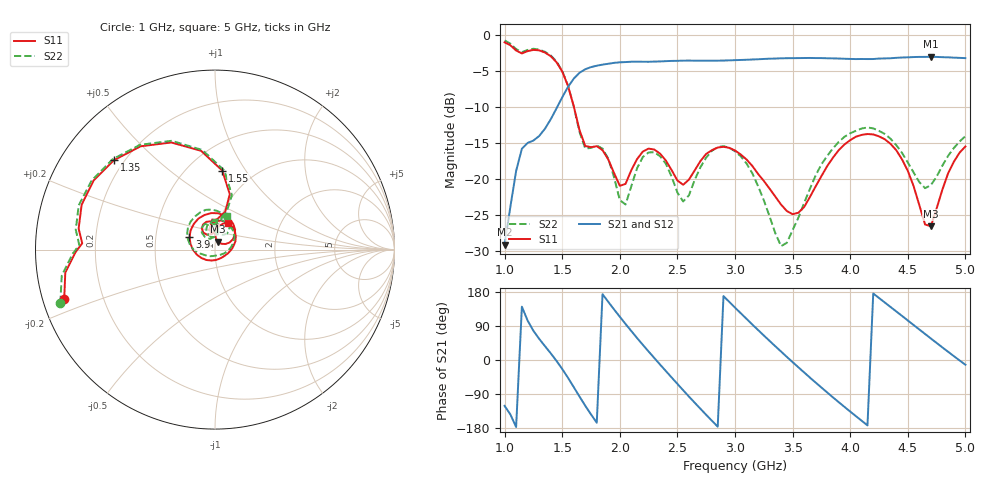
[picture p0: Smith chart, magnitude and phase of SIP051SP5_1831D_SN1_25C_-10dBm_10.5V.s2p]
# GHz  S  dB  R  50
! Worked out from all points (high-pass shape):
!   81 points, 1 GHz to 5 GHz, reference 50 ohm
!   highest |S21| = -3.07 dB at 4.7 GHz (marker M1); lowest = -29.2 dB at 1 GHz (marker M2)
!   |S21| within 3 dB of the highest: 1.602 GHz to end of sweep
!   lowest |S11| = -26.6 dB at 4.7 GHz (marker M3), VSWR 1.10, Z = 51.5 + j4.52 ohm
!   |S11| at or under -10 dB: 1.601 GHz to end of sweep
!   |S22| runs from -29.3 to -0.8 dB; largest |S21 - S12| = 0.0026
!   S11 on the Smith chart (normalised r, x): 1 GHz: 0.06, -0.16; 1.35 GHz: 0.16, +0.37; 1.55 GHz: 0.72, +0.79; 3.9 GHz: 0.74, +0.11; 5 GHz: 1.10, +0.34
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1  -1.06 -161.7  -29.15 -121.1  -29.17 -121.1  -0.81 -161.0
1.15  -2.61 177.3  -15.82 140.7  -15.86 140.8  -2.42 178.1
1.35  -2.48 138.4  -13.06 36.7  -13.05 36.6  -2.38 138.5
1.55  -7.09 84.7  -7.26 -46.8  -7.25 -46.7  -7.06 83.3
1.7  -15.44 86.2  -4.80 -120.7  -4.81 -120.6  -15.79 86.8
1.85  -16.02 91.6  -4.16 173.7  -4.15 173.8  -15.80 89.0
2.05  -20.70 117.4  -3.80 95.0  -3.81 95.0  -23.56 115.0
2.2  -16.22 115.8  -3.76 40.0  -3.75 40.0  -16.97 121.6
2.35  -16.51 91.1  -3.71 -12.1  -3.72 -12.1  -16.87 93.1
2.6  -20.11 102.9  -3.60 -96.4  -3.61 -96.3  -22.29 108.8
2.8  -16.03 87.5  -3.61 -160.4  -3.61 -160.4  -16.10 98.8
3  -16.06 50.3  -3.54 138.4  -3.53 138.4  -16.17 55.6
3.2  -19.31 13.5  -3.42 79.2  -3.41 79.4  -21.00 7.9
3.4  -23.58 -28.0  -3.28 22.2  -3.28 22.2  -29.34 -71.4
3.55  -24.70 -85.0  -3.25 -19.2  -3.24 -19.2  -25.40 -139.8
3.7  -21.05 -147.7  -3.25 -59.6  -3.25 -59.4  -19.53 -174.3
3.9  -16.02 154.2  -3.31 -111.1  -3.33 -111.2  -14.89 149.2
4.15  -13.79 95.6  -3.38 -172.5  -3.37 -172.3  -12.88 103.0
4.35  -15.15 54.3  -3.27 139.9  -3.28 139.9  -14.44 69.6
4.55  -20.99 25.8  -3.11 92.4  -3.12 92.5  -19.10 53.4
4.7  -26.58 69.0  -3.07 56.8  -3.07 56.9  -20.88 84.7
5  -15.51 64.1  -3.26 -12.5  -3.26 -12.5  -14.08 69.7
